(* Logix 5000 AddOnInstructionDefinition export AMCI_3204_AOP_Manual_Move_CCW; software revision 20.03 *)

ADD_ON_INSTRUCTION AMCI_3204_AOP_Manual_Move_CCW   (* revision 1.0, vendor AMCI, ExecuteEnableInFalse *)
VAR_INPUT
   axis_status_bits : INT; {required}
   channel_number : INT; {required}
   _0_normal_1_S_Curve_Acceleration : BOOL;
   _0_Triangular_1_Trapezoidal_S_Curve : BOOL;
   Programmed_speed : DINT; {required}
   Acceleration : DINT; {required}
   Deceleration : DINT; {required}
END_VAR
VAR_IN_OUT
   AMCI_3204_output_data : AM:1756_3204:O:0; {required}
END_VAR
VAR_OUTPUT
   EN : BOOL; {access Read Only, visible}
   Manual_Move_CCW_occurring : BOOL; {access Read Only, visible}
   ER : BOOL; {access Read Only, visible}
END_VAR
VAR
   command_data_block : DINT[8]; {access None}
END_VAR

ROUTINE EnableInFalse   (* ladder *)
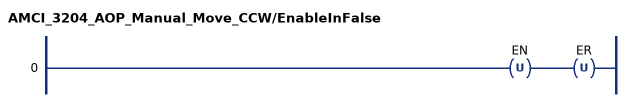
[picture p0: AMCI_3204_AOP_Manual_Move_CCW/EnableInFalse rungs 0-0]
   0: OTU(EN)OTU(ER);
END_ROUTINE

ROUTINE Logic   (* ladder *)
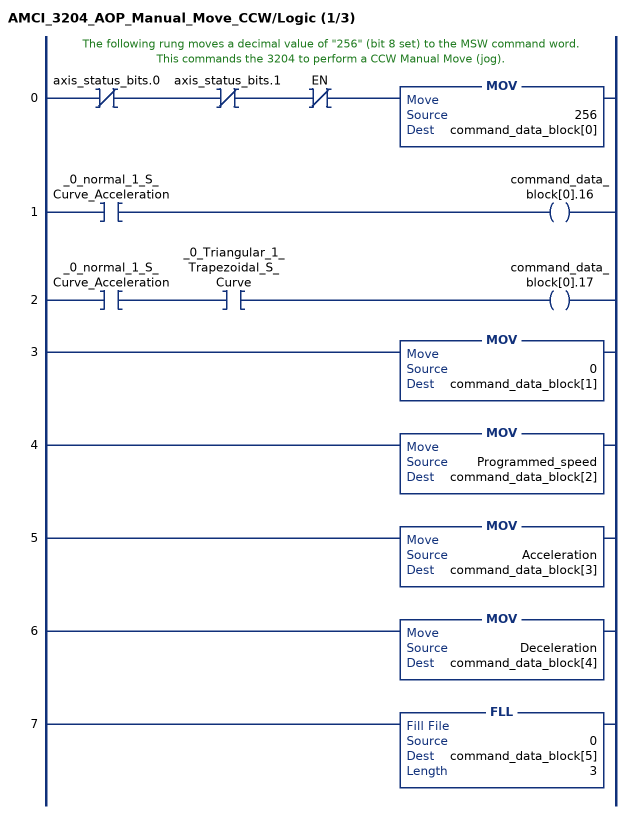
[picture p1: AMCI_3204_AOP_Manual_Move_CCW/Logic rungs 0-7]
   // The following rung moves a decimal value of "256" (bit 8 set) to the MSW command word.  This commands the 3204 to perform a CCW Manual Move (jog).
   0: XIO(axis_status_bits.0)XIO(axis_status_bits.1)XIO(EN)MOV(256,command_data_block[0]);
   1: XIC(_0_normal_1_S_Curve_Acceleration)OTE(command_data_block[0].16);
   2: XIC(_0_normal_1_S_Curve_Acceleration)XIC(_0_Triangular_1_Trapezoidal_S_Curve)OTE(command_data_block[0].17);
   3: MOV(0,command_data_block[1]);
   4: MOV(Programmed_speed,command_data_block[2]);
   5: MOV(Acceleration,command_data_block[3]);
   6: MOV(Deceleration,command_data_block[4]);
   7: FLL(0,command_data_block[5],3);
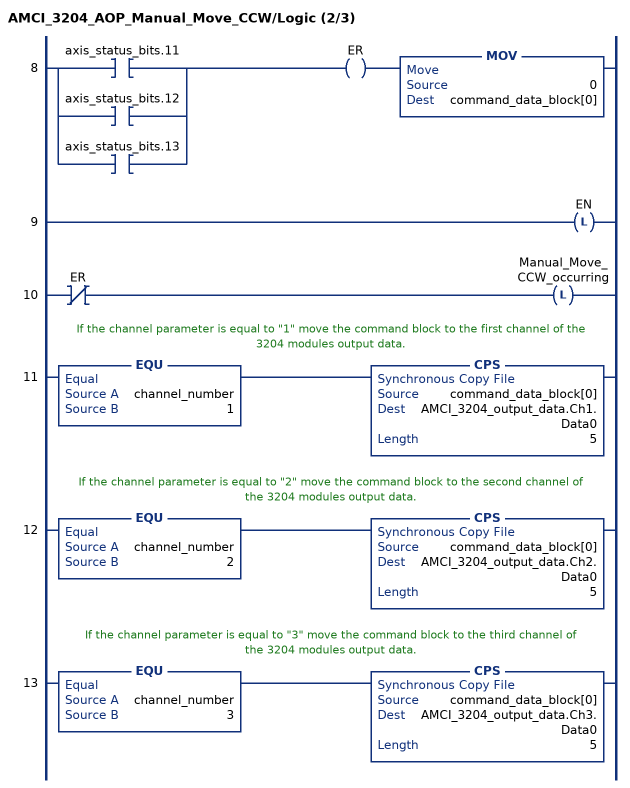
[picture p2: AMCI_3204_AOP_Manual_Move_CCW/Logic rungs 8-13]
   8: [XIC(axis_status_bits.11) ,XIC(axis_status_bits.12) ,XIC(axis_status_bits.13) ]OTE(ER)MOV(0,command_data_block[0]);
   9: OTL(EN);
   10: XIO(ER)OTL(Manual_Move_CCW_occurring);
   // If the channel parameter is equal to "1" move the command block to the first channel of the 3204 modules output data.
   11: EQU(channel_number,1)CPS(command_data_block[0],AMCI_3204_output_data.Ch1.Data0,5);
   // If the channel parameter is equal to "2" move the command block to the second channel of the 3204 modules output data.
   12: EQU(channel_number,2)CPS(command_data_block[0],AMCI_3204_output_data.Ch2.Data0,5);
   // If the channel parameter is equal to "3" move the command block to the third channel of the 3204 modules output data.
   13: EQU(channel_number,3)CPS(command_data_block[0],AMCI_3204_output_data.Ch3.Data0,5);
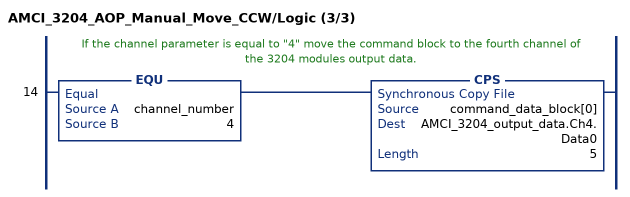
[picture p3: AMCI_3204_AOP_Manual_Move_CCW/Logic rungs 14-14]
   // If the channel parameter is equal to "4" move the command block to the fourth channel of the 3204 modules output data.
   14: EQU(channel_number,4)CPS(command_data_block[0],AMCI_3204_output_data.Ch4.Data0,5);
END_ROUTINE
END_ADD_ON_INSTRUCTION
